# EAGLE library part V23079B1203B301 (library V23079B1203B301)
DPDT-NO/NC Through Hole Latching Relay, 2 A, 12V dc Source: Datasheet
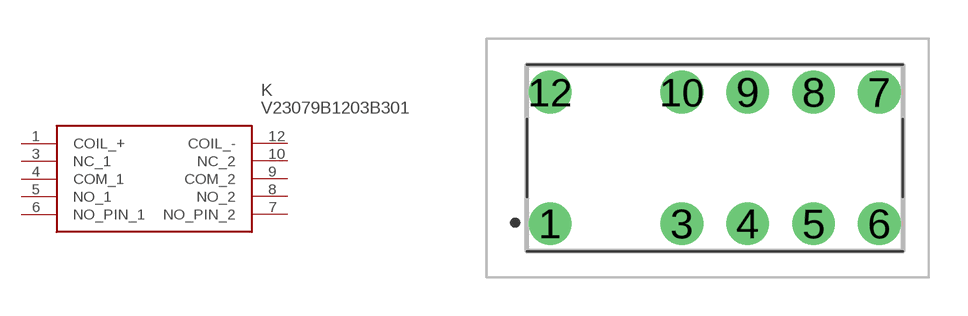
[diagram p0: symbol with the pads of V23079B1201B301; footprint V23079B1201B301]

Designator prefix K

## V23079B1203B301 (Description: DPDT-NO/NC Through Hole Latching Relay, 2 A, 12V dc; Height: 9mm; Manufacturer_Name: TE Connectivity; Manufacturer_Part_Number: V23079B1203B301; Mouser_Part_Number: 655-V23079B1203B301; Mouser_Price-Stock: https://www.mouser.co.uk/ProductDetail/TE-Connectivity-PB/V23079B1203B301?qs=CizG3IxbuFPu%2FPkh3nhEBw%3D%3D)  [V23079B1201B301]
1  COIL_+
3  NC_1
4  COM_1
5  NO_1
6  NO_PIN_1
7  NO_PIN_2
8  NO_2
9  COM_2
10  NC_2
12  COIL_-

## Footprint V23079B1201B301 (pad centres in mm)
V23079 2 coil
drill 1.1 pad 1.65: 1 -6.35,-2.54; 3 -1.27,-2.54; 4 1.27,-2.54; 5 3.81,-2.54; 6 6.35,-2.54; 7 6.35,2.54; 8 3.81,2.54; 9 1.27,2.54; 10 -1.27,2.54; 12 -6.35,2.54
